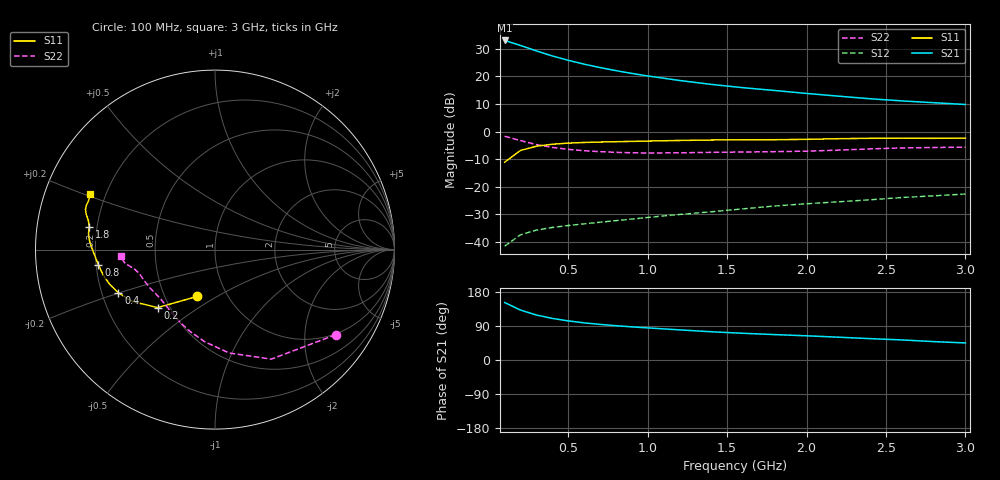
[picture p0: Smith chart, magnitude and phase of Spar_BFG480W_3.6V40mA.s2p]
! Filename: 3_640BFG480.001
! Title: BFG480W
! Bias: Vce=3.6V; Ic=40mA
! Company: NXP Semiconductors NL
! User: Quality&Reliability T&D
! Measure time: 10 Nov 1999 / 11:59:46
#  MHz  S  MA  R 50
! Freq  S11  S21  S12  S22  :
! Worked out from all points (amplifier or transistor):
!   20 points, 100 MHz to 3 GHz, reference 50 ohm
!   highest |S21| = 33.0 dB at 100 MHz (marker M1)
!   |S21| within 3 dB of that: start of sweep to 259.9 MHz
!   unconditionally stable (mu >= 1): 1.052 GHz to end of sweep
!   at 400 MHz: K = 0.58, MSG = 31.1 dB, |S12| = -34.8 dB
!   at 1.2 GHz: K = 1.04, MAG = 23.1 dB, |S12| = -30.1 dB
!   at 3 GHz: K = 1.07, MAG = 14.7 dB, |S12| = -22.7 dB
!   S11 on the Smith chart (normalised r, x): 100 MHz: 0.72, -0.41; 200 MHz: 0.43, -0.35; 400 MHz: 0.27, -0.20; 800 MHz: 0.21, -0.06; 1.8 GHz: 0.17, +0.09; 3 GHz: 0.14, +0.21
100  0.2787 -110.7  44.92 151.8  0.008355 66.3  0.8227 -35.2
200  0.4546 -134.7  36.46 131.7  0.01343 55.7  0.6862 -62.8
300  0.5429 -147.8  29.02 118.7  0.01633 51.0  0.5812 -82.3
400  0.5895 -155.8  23.53 109.8  0.01827 49.7  0.5162 -96.5
500  0.6173 -161.7  19.63 103.2  0.01978 50.1  0.4759 -107.2
600  0.6344 -166.0  16.7 98.1  0.02124 51.3  0.45 -115.5
700  0.6458 -169.6  14.5 94.0  0.02269 53.2  0.4323 -122.0
800  0.655 -172.6  12.75 90.5  0.02428 55.3  0.4203 -127.5
900  0.6637 -175.2  11.34 87.5  0.02587 57.5  0.4129 -132.3
1000  0.6727 -177.6  10.22 84.7  0.02771 59.3  0.4094 -136.6
1200  0.69 178.4  8.453 79.5  0.03139 62.5  0.4121 -143.8
1400  0.7032 175.5  7.169 74.5  0.03512 64.9  0.4201 -149.2
1600  0.7103 172.8  6.252 70.5  0.03969 67.2  0.4259 -153.3
1800  0.712 169.8  5.558 67.0  0.04474 68.9  0.4324 -157.4
2000  0.7228 167.3  4.919 63.9  0.04908 70.5  0.4418 -162.2
2200  0.7427 164.8  4.391 60.2  0.05332 71.2  0.4609 -166.3
2400  0.7553 162.8  3.938 56.4  0.05795 71.4  0.4855 -169.2
2600  0.7583 161.0  3.599 53.0  0.06375 71.3  0.5051 -171.0
2800  0.7553 158.7  3.34 48.5  0.06838 70.5  0.5147 -173.0
3000  0.7605 156.0  3.1 45.0  0.07364 70.1  0.5224 -176.1
